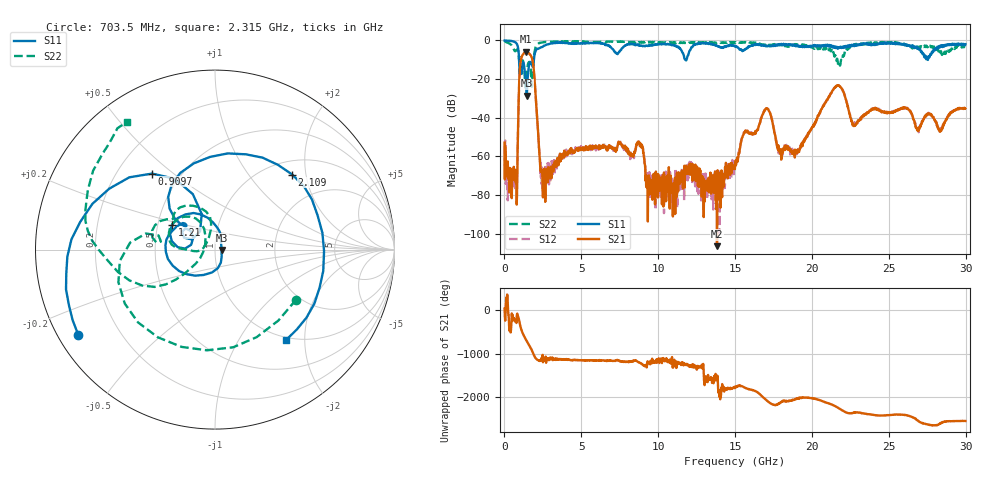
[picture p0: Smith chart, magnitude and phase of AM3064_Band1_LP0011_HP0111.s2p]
# Hz S DB R 50.0
!freq dBS11 angS11 dBS21 angS21 dBS12 angS12 dBS22 angS22
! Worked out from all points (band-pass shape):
!   1600 points, 10 MHz to 29.98 GHz, reference 50 ohm
!   highest |S21| = -5.83 dB at 1.416 GHz (marker M1); lowest = -106.5 dB at 13.82 GHz (marker M2)
!   |S21| within 3 dB of the highest: 1.108 GHz to 1.774 GHz (666.5 MHz wide, 46.3 % of centre)
!   lowest |S11| = -28.6 dB at 1.453 GHz (marker M3), VSWR 1.08, Z = 53.8 - j0.179 ohm
!   |S11| at or under -10 dB: 949.3 MHz to 1.914 GHz (964.8 MHz wide, 67.4 % of centre); 11.75 GHz to 11.84 GHz (87.27 MHz wide, 0.74 % of centre); 27.52565 GHz to 27.54652 GHz (20.87 MHz wide, 0.0758 % of centre)
!   |S22| runs from -24.5 to -0.3 dB; largest |S21 - S12| = 0.0062
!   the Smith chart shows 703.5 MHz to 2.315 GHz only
!   S11 on the Smith chart (normalised r, x): 703.5 MHz: 0.06, -0.29; 909.7 MHz: 0.35, +0.42; 1.21 GHz: 0.59, +0.18; 2.109 GHz: 1.28, +1.67; 2.315 GHz: 0.95, -1.63
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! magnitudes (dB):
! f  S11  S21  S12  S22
! 10 MHz  0.0  -52.9  -54.5  -0.3
! 703.5 MHz  -0.9  -72.4  -71.6  -5.5
! 909.7 MHz  -5.2  -36.0  -36.0  -6.5
! 1.21 GHz  -11.2  -7.2  -7.1  -10.6
! 1.416 GHz  -23.0  -5.8  -5.8  -19.9
! 1.453 GHz  -28.6  -5.9  -5.8  -16.8
! 1.828 GHz  -13.5  -10.4  -10.4  -17.7
! 2.109 GHz  -4.4  -38.1  -38.0  -2.3
! 2.315 GHz  -3.9  -63.6  -61.7  -1.3
! 2.597 GHz  -2.7  -66.3  -68.9  -0.9
! 5.015 GHz  -1.4  -56.5  -56.1  -0.6
! 8.801 GHz  -2.7  -54.6  -52.9  -0.9
! 10 GHz  -2.0  -69.2  -75.9  -0.9
! 13.82 GHz  -2.7  -106.5  -69.1  -1.0
! 15 GHz  -3.1  -63.6  -62.6  -1.3
! 17.01 GHz  -3.1  -35.2  -35.5  -2.5
! 17.97 GHz  -2.4  -58.8  -57.4  -2.1
! 19.99 GHz  -3.2  -45.4  -45.6  -3.4
! 21.66 GHz  -3.8  -23.4  -23.4  -10.0
! 22.75 GHz  -3.0  -44.0  -44.2  -2.0
! 25 GHz  -1.1  -37.1  -37.1  -1.0
! 29.98 GHz  -1.9  -35.2  -35.2  -3.2
